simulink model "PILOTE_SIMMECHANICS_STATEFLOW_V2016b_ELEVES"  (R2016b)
settings: Solver=ode45  StartTime=0  StopTime=30  MaxStep=0.05  RelTol=1e-3  EnableMultiTasking=on
undefined symbols (not defined in the file): Bati, coulisseau, deg, kg, m, N, PILOTE_SIMULINK, rad, RootGround, RootPart, s
libraries: mblibv1 x16

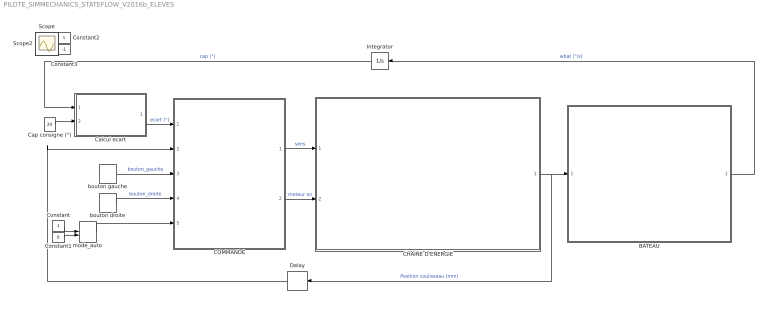
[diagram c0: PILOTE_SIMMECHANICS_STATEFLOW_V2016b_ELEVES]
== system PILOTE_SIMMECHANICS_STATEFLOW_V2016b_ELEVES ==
  BATEAU : Subsystem
  CHAINE D'ENERGIE : Subsystem
  COMMANDE : Stateflow chart  TreatAsAtomicUnit=on
  Calcul ecart : MATLAB Function  TreatAsAtomicUnit=on
  Cap consigne (°) : Constant  Value=20
  Constant : Constant
  Constant1 : Constant  Value=0
  Constant2 : Constant
  Constant3 : Constant  Value=-1
  Delay : Delay  DelayLength=1  SampleTime=0.05
  Integrator : Integrator
  bouton droite : DiscretePulseGenerator  PulseType=Time based  Period=30  PulseWidth=40  PhaseDelay=15
  bouton gauche : DiscretePulseGenerator  PulseType=Time based  Period=30  PulseWidth=40  PhaseDelay=1
  mode_auto : ManualSwitch  CurrentSetting=0
  Scope : Scope
  Scope2 : Scope
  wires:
  Constant/1 -> mode_auto/1
  Constant1/1 -> mode_auto/2
  bouton gauche/1 -> COMMANDE/3(bouton_gauche)  "bouton_gauche"
  bouton droite/1 -> COMMANDE/4(bouton_droite)  "bouton_droite"
  mode_auto/1 -> COMMANDE/5(mode_auto)
  COMMANDE/1(sens_rotation) -> CHAINE D'ENERGIE/1(sens)  "sens"
  COMMANDE/2(moteur_on) -> CHAINE D'ENERGIE/2(moteur_on)  "moteur on"
  BATEAU/1(Out1) -> Integrator/1  "wbat (°/s)"
  Calcul ecart/1(ecart) -> COMMANDE/1(ecart_cap)  "ecart (°)"
  Cap consigne (°)/1 -> Calcul ecart/2(cap_consigne)
  CHAINE D'ENERGIE/1(Pos_coul) -> Delay/1, BATEAU/1(In1)  "Position coulisseau (mm)"
  Integrator/1 -> Calcul ecart/1(cap_mesure)  "cap (°)"
  Constant2/1 -> ?
  Constant3/1 -> ?
  Delay/1 -> COMMANDE/2(pos_coul)

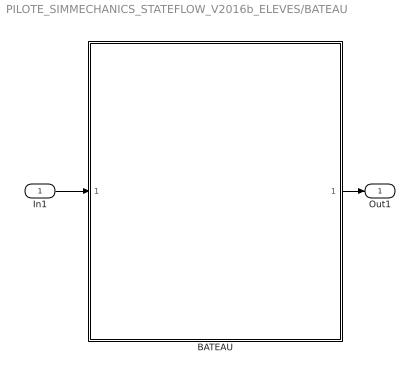
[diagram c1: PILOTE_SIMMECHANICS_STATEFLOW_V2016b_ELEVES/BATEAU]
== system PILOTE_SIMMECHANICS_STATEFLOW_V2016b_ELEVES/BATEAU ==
  In1 : Inport
  BATEAU : MATLAB Function  TreatAsAtomicUnit=on
  Out1 : Outport
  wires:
  In1/1 -> BATEAU/1(pos)
  BATEAU/1(wbat) -> Out1/1

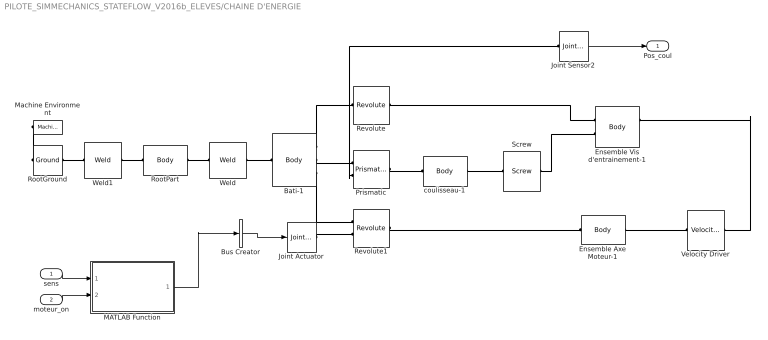
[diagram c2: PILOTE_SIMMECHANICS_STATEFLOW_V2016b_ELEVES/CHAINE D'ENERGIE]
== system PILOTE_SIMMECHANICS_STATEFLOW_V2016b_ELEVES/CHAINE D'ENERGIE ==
  sens : Inport
  moteur_on : Inport  Port=2
  Bati-1 : mblibv1/Bodies/Body  LConnTagsString=CS2  RConnTagsString=CS3|CS4|CS5  UpdateFromCAD=on  PMImportedID=Bati-1  DialogClass=MechanicalBodyBlock  Mass=0.275117  MassUnits=kg  InertiaUnits=kg*m^2  Inertia=[0.00487661,-3.37196e-06,-0.000236406;-3.37196e-06,0.00504829,7.5779e-05;-0.000236406,7.5779e-05,0.000251799]  Shape=Cylinder  ShapeDims=[1 1]  ShapeUnits=m  ShapeUse=false  Density=1  DensityUnits=kg/m^3  DensityUse=false  GraphicsMode=GFXFILE  GraphicsFileName=PILOTE_SIMULINK - Bati-1.STL  BodyColorSelMode=COLORPALETTE  BodyColor=[0.75294 0.75294 0.75294]  AttachedToCS=CS1  CG=Right$CG$[0.280395 0.00767074 -0.0225996]$WORLD$WORLD$m$[0 0 1;1 0 0;0 1 0]$3x3 Transform$rad$WORLD$false$Bati-1::CG(AUTOGEN)  WorkingFrames=Right$CS1$[0 0 0]$WORLD$WORLD$m$[0 0 1;1 0 0;0 1 0]$3x3 Transform$rad$WORLD$false$Bati-1::CS1(AUTOGEN)#Left$CS2$[0.280395 0.00767074 -0.0225996]$WORLD$WORLD$m$[1 0 0;0 1 0;0 0 1]$3x3 Transform$rad$WORLD$true$Bati-1:-:PILOTE_SIMULINK/RootPart::Bati-1(AUTOGEN)#Right$CS3$[0.341 0 -0.015]$WORLD$WORLD$m$[1 0 0;0 1 0;0 0 1]$3x3 Transform$rad$WORLD$true$Bati-1:-:Ensemble Vis d'entrainement-1::Bati-1(AUTO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  CGPos=[0.280395 0.00767074 -0.0225996]  CGRot=[0 0 1;1 0 0;0 1 0]  CS0Pos=[]  CS0Rot=[]  CS1Pos=[0 0 0]  CS1Rot=[0 0 1;1 0 0;0 1 0]  CS2Pos=[0.280395 0.00767074 -0.0225996]  CS2Rot=[1 0 0;0 1 0;0 0 1]  CS3Pos=[0.341 0 -0.015]  CS3Rot=[1 0 0;0 1 0;0 0 1]  CS4Pos=[-0.00290422 0 -0.015]  CS4Rot=[1 0 0;0 1 0;0 0 1]  CS5Pos=[0.371 0.0399019 -0.0121998]  CS5Rot=[1 0 0;0 1 0;0 0 1]  CS6Pos=[0.341 0 -0.015]  CS6Rot=[1 0 0;0 1 0;0 0 1]  CS7Pos=[]  CS7Rot=[]  CS8Pos=[]  CS8Rot=[]  CS9Pos=[]  CS9Rot=[]  CS10Pos=[]  CS10Rot=[]  CS11Pos=[]  CS11Rot=[]  CS12Pos=[]  CS12Rot=[]  CS13Pos=[]  CS13Rot=[]  CS14Pos=[]  CS14Rot=[]  CS15Pos=[]  CS15Rot=[]  CS16Pos=[]  CS16Rot=[]  CS17Pos=[]  CS17Rot=[]  CS18Pos=[]  CS18Rot=[]  CS19Pos=[]  CS19Rot=[]  CS20Pos=[]  CS20Rot=[]
  Bus Creator : BusCreator  Inputs=3
  Ensemble Axe Moteur-1 : mblibv1/Bodies/Body  LConnTagsString=CS2  RConnTagsString=CS1  UpdateFromCAD=on  PMImportedID=Ensemble Axe Moteur-1  DialogClass=MechanicalBodyBlock  Mass=0.330709  MassUnits=kg  InertiaUnits=kg*m^2  Inertia=[5e-05,0,0;0,5e-05,0;0,0,5e-05]  Shape=Cylinder  ShapeDims=[1 1]  ShapeUnits=m  ShapeUse=false  Density=1  DensityUnits=kg/m^3  DensityUse=false  GraphicsMode=GFXFILE  GraphicsFileName=PILOTE_SIMULINK - Ensemble Axe Moteur-1.STL  BodyColorSelMode=COLORPALETTE  BodyColor=[1 0 1]  AttachedToCS=CS1  CG=Right$CG$[0.388245 0.0399019 -0.0121998]$WORLD$WORLD$m$[-1 0 0;0 0.998629 -0.0523416;0 -0.0523416 -0.998629]$3x3 Transform$rad$WORLD$false$Ensemble Axe Moteur-1::CG(AUTOGEN)  WorkingFrames=Right$CS1$[0.373663 0.0782415 -0.0142093]$WORLD$WORLD$m$[-1 0 0;0 0.998629 -0.0523416;0 -0.0523416 -0.998629]$3x3 Transform$rad$WORLD$true$Ensemble Axe Moteur-1::CS1(AUTOGEN)#Left$CS2$[0.371 0.0399019 -0.0121998]$WORLD$WORLD$m$[1 0 0;0 1 0;0 0 1]$3x3 Transform$rad$WORLD$true$Bati-1:-:Ensemble Axe Moteur-1::Ensemble Axe Moteur-1(AUTOGEN)  CGPos=[0.388245 0.0399019 -0.0121998]  CGRot=[-1 0 0;0 0.998629 -0.0523416;0 -0.0523416 -0.998629]  CS0Pos=[]  CS0Rot=[]  CS1Pos=[0.373663 0.0782415 -0.0142093]  CS1Rot=[-1 0 0;0 0.998629 -0.0523416;0 -0.0523416 -0.998629]  CS2Pos=[0.371 0.0399019 -0.0121998]  CS2Rot=[1 0 0;0 1 0;0 0 1]  CS3Pos=[]  CS3Rot=[]  CS4Pos=[]  CS4Rot=[]  CS5Pos=[]  CS5Rot=[]  CS6Pos=[]  CS6Rot=[]  CS7Pos=[]  CS7Rot=[]  CS8Pos=[]  CS8Rot=[]  CS9Pos=[]  CS9Rot=[]  CS10Pos=[]  CS10Rot=[]  CS11Pos=[]  CS11Rot=[]  CS12Pos=[]  CS12Rot=[]  CS13Pos=[]  CS13Rot=[]  CS14Pos=[]  CS14Rot=[]  CS15Pos=[]  CS15Rot=[]  CS16Pos=[]  CS16Rot=[]  CS17Pos=[]  CS17Rot=[]  CS18Pos=[]  CS18Rot=[]  CS19Pos=[]  CS19Rot=[]  CS20Pos=[]  CS20Rot=[]
  Ensemble Vis d'entrainement-1 : mblibv1/Bodies/Body  LConnTagsString=CS2|CS3  RConnTagsString=CS1|CS4  UpdateFromCAD=on  PMImportedID=Ensemble Vis d'entrainement-1  DialogClass=MechanicalBodyBlock  Mass=0.163769  MassUnits=kg  InertiaUnits=kg*m^2  Inertia=[0.00190405,1.37845e-10,-2.6424e-08;1.37845e-10,0.00190406,-8.48302e-09;-2.6424e-08,-8.48302e-09,4.54904e-06]  Shape=Cylinder  ShapeDims=[1 1]  ShapeUnits=m  ShapeUse=false  Density=1  DensityUnits=kg/m^3  DensityUse=false  GraphicsMode=GFXFILE  GraphicsFileName=PILOTE_SIMULINK - Ensemble Vis d'entrainement-1.STL  BodyColorSelMode=COLORPALETTE  BodyColor=[1 0 0]  AttachedToCS=CS1  CG=Right$CG$[0.18733 -5.19925e-07 -0.0149984]$WORLD$WORLD$m$[0 0 -1;-0.606632 -0.794983 0;-0.794983 0.606632 0]$3x3 Transform$rad$WORLD$false$Ensemble Vis d'entrainement-1::CG(AUTOGEN)  WorkingFrames=Right$CS1$[0.361 0 -0.015]$WORLD$WORLD$m$[0 0 -1;-0.606632 -0.794983 0;-0.794983 0.606632 0]$3x3 Transform$rad$WORLD$true$Ensemble Vis d'entrainement-1::CS1(AUTOGEN)#Left$CS2$[0.341 0 -0.015]$WORLD$WORLD$m$[1 0 0;0 1 0;0 0 1]$3x3 Transform$rad$WORLD$true$Bati-1:-:Ensemble Vis d'entrainement-1::Ensemble Vis d'entrainement-1(AUTOGEN)#Right$CS4$[0.341 0 -0.015]$WORLD$WORLD$m$[1 0 0;0 1 0;0 0 1]$3x3 T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  CGPos=[0.18733 -5.19925e-07 -0.0149984]  CGRot=[0 0 -1;-0.606632 -0.794983 0;-0.794983 0.606632 0]  CS0Pos=[]  CS0Rot=[]  CS1Pos=[0.361 0 -0.015]  CS1Rot=[0 0 -1;-0.606632 -0.794983 0;-0.794983 0.606632 0]  CS2Pos=[0.341 0 -0.015]  CS2Rot=[1 0 0;0 1 0;0 0 1]  CS3Pos=[0.0706 0 -0.015]  CS3Rot=[1 0 0;0 1 0;0 0 1]  CS4Pos=[0.341 0 -0.015]  CS4Rot=[1 0 0;0 1 0;0 0 1]  CS5Pos=[]  CS5Rot=[]  CS6Pos=[]  CS6Rot=[]  CS7Pos=[]  CS7Rot=[]  CS8Pos=[]  CS8Rot=[]  CS9Pos=[]  CS9Rot=[]  CS10Pos=[]  CS10Rot=[]  CS11Pos=[]  CS11Rot=[]  CS12Pos=[]  CS12Rot=[]  CS13Pos=[]  CS13Rot=[]  CS14Pos=[]  CS14Rot=[]  CS15Pos=[]  CS15Rot=[]  CS16Pos=[]  CS16Rot=[]  CS17Pos=[]  CS17Rot=[]  CS18Pos=[]  CS18Rot=[]  CS19Pos=[]  CS19Rot=[]  CS20Pos=[]  CS20Rot=[]
  Joint Actuator : mblibv1/Sensors &  Actuators/Joint Actuator  UpdateFromCAD=off  PhysicalDomain=Mechanical  PortType=blob  ActuationStyle=Motion  AngleUnits=rad  ArcVelocityUnits=rad/s  ArcAccelerationUnits=rad/s^2  CoordPositionUnits=m  VelocityUnits=m/s  AccelerationUnits=m/s^2  ForceUnits=N  TorqueUnits=N*m  ActiveIO=on  Width=3  DialogClass=MechanicalActuatorBlock  Primitive=R1  ReferenceFrame=Absolute (World)
  Joint Sensor2 : mblibv1/Sensors &  Actuators/Joint Sensor  UpdateFromCAD=off  PhysicalDomain=Mechanical  PortType=blob  Muxed=off  Pose=off  Angle=off  AngleUnits=deg  ArcVelocity=off  ArcVelocityUnits=deg/s  ArcAcceleration=off  ArcAccelerationUnits=deg/s^2  CoordPosition=on  CoordPositionUnits=mm  Velocity=off  VelocityUnits=m/s  Acceleration=off  AccelerationUnits=m/s^2  Quaternion=on  QuaternionDT=off  QuaternionDDT=off  QuaternionUnits=off  OutputVector=[1]  ActiveIO=on  Width=1  DialogClass=MechanicalSensorBlock  Primitive=P1  Force=off  ForceUnits=N  Torque=on  TorqueUnits=N*m  ReferenceFrame=Absolute (World)  ReactionSensedSide=Base  ReactionReferenceFrame=Absolute (World)  ReactionForce=off  ReactionForceUnits=N  ReactionMoment=off  ReactionMomentUnits=N*m
  MATLAB Function : MATLAB Function  TreatAsAtomicUnit=on
  Machine Environment : mblibv1/Bodies/Machine Environment  PortType=env  PhysicalDomain=Mechanical  DialogTemplateClass=MECH.MachineEnvironment  SyncWhenCopied=off  Gravity=[0 -9.81 0]  GravityUnits=m/s^2  GravityAsSignal=off  Dimensionality=Auto-detect  AnalysisType=Forward dynamics  LinearAssemblyTolerance=1e-3  LinearAssemblyToleranceUnits=m  AngularAssemblyTolerance=1e-3  AngularAssemblyToleranceUnits=rad  ConstraintSolverType=Stabilizing  ConstraintRelTolerance=1e-4  ConstraintAbsTolerance=1e-4  UseRobustSingularityHandling=off  RedundancyAnalysisToleranceType=Automatically select tolerance  RedundancyAnalysisTolerance=1e-14  StatePerturbationType=Fixed  PerturbationSize=1e-5  VisualizeMachine=on  BodyVisualizationType=Use model default body geometries  BodyColorSelMode=Use model default  DefaultBodyColor=[1 0 0]
  Prismatic : mblibv1/Joints/Prismatic  LConnTagsString=__newl0|SA1  RConnTagsString=__newr0  UpdateFromCAD=on  PMImportedID=Bati-1:-:coulisseau-1  NumSAPorts=1  CutJoint=off  MarkAsCut=off  Primitives=prismatic  PrimitiveProps=P1$World$[-1,0,0]$prismatic  DialogClass=JointBlock  P1Axis=[-1,0,0]
  Revolute : mblibv1/Joints/Revolute  LConnTagsString=__newl0  RConnTagsString=__newr0  UpdateFromCAD=on  PMImportedID=Bati-1:-:Ensemble Vis d'entrainement-1  NumSAPorts=0  CutJoint=off  MarkAsCut=off  Primitives=prismatic  PrimitiveProps=R1$World$[1,0,0]$revolute  DialogClass=JointBlock  R1Axis=[1,0,0]
  Revolute1 : mblibv1/Joints/Revolute  LConnTagsString=__newl0|SA1  RConnTagsString=__newr0  UpdateFromCAD=on  PMImportedID=Bati-1:-:Ensemble Axe Moteur-1  NumSAPorts=1  CutJoint=off  MarkAsCut=off  Primitives=prismatic  PrimitiveProps=R1$World$[-1,0,0]$revolute  DialogClass=JointBlock  R1Axis=[-1,0,0]
  RootGround : mblibv1/Bodies/Ground  UpdateFromCAD=on  PMImportedID=RootGround  LeftPortType=env  RightPortType=workingframe  PhysicalDomain=Mechanical  DialogClass=GroundBlock  CoordPosition=[0.246549,0.0167324,-0.0162514]  CoordPositionUnits=m  StateVectorMgrId=2  MachineId=[3 0]  ShowEnvPort=on  ParameterChecksum=[441952517, 4021082612, 3603074577, 143967490]  TopologyChecksum=[1489896608, 3478853089, 1162583120, 1816670376]
  RootPart : mblibv1/Bodies/Body  LConnTagsString=CS3  RConnTagsString=CS2  UpdateFromCAD=on  PMImportedID=PILOTE_SIMULINK/RootPart  DialogClass=MechanicalBodyBlock  Mass=0  MassUnits=kg  InertiaUnits=kg*m^2  Inertia=[0,0,0;0,0,0;0,0,0]  Shape=Cylinder  ShapeDims=[1 1]  ShapeUnits=m  ShapeUse=false  Density=1  DensityUnits=kg/m^3  DensityUse=false  GraphicsMode=MACHINE_DEFAULT  BodyColorSelMode=MACHINE_DEFAULT  BodyColor=[1;0;0]  AttachedToCS=CS1  CG=Right$CG$[0.246549 0.0167324 -0.0162514]$WORLD$WORLD$m$[1 0 0;0 1 0;0 0 1]$3x3 Transform$rad$WORLD$false$PILOTE_SIMULINK/RootPart::CG(AUTOGEN)  WorkingFrames=Right$CS1$[0 0 0]$WORLD$WORLD$m$[1 0 0;0 1 0;0 0 1]$3x3 Transform$rad$WORLD$false$PILOTE_SIMULINK/RootPart::CS1(AUTOGEN)#Right$CS2$[0.280395 0.00767074 -0.0225996]$WORLD$WORLD$m$[1 0 0;0 1 0;0 0 1]$3x3 Transform$rad$WORLD$true$Bati-1:-:PILOTE_SIMULINK/RootPart::PILOTE_SIMULINK/RootPart(AUTOGEN)#Left$CS3$[0.246549 0.0167324 -0.0162514]$WORLD$WORLD$m$[1 0 0;0 1 0;0 0 1]$3x3 Transform$rad$WORLD$true$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  CGPos=[0.246549 0.0167324 -0.0162514]  CGRot=[1 0 0;0 1 0;0 0 1]  CS0Pos=[]  CS0Rot=[]  CS1Pos=[0 0 0]  CS1Rot=[1 0 0;0 1 0;0 0 1]  CS2Pos=[0.280395 0.00767074 -0.0225996]  CS2Rot=[1 0 0;0 1 0;0 0 1]  CS3Pos=[0.246549 0.0167324 -0.0162514]  CS3Rot=[1 0 0;0 1 0;0 0 1]  CS4Pos=[]  CS4Rot=[]  CS5Pos=[]  CS5Rot=[]  CS6Pos=[]  CS6Rot=[]  CS7Pos=[]  CS7Rot=[]  CS8Pos=[]  CS8Rot=[]  CS9Pos=[]  CS9Rot=[]  CS10Pos=[]  CS10Rot=[]  CS11Pos=[]  CS11Rot=[]  CS12Pos=[]  CS12Rot=[]  CS13Pos=[]  CS13Rot=[]  CS14Pos=[]  CS14Rot=[]  CS15Pos=[]  CS15Rot=[]  CS16Pos=[]  CS16Rot=[]  CS17Pos=[]  CS17Rot=[]  CS18Pos=[]  CS18Rot=[]  CS19Pos=[]  CS19Rot=[]  CS20Pos=[]  CS20Rot=[]
  Screw : mblibv1/Joints/Screw  LConnTagsString=__newl0  RConnTagsString=__newr0  UpdateFromCAD=off  NumSAPorts=0  CutJoint=off  MarkAsCut=off  Primitives=prismatic  PrimitiveProps=R1$World$[1 0 0]$revolute  DialogClass=ScrewJointBlock  Pitch=3  Units=mm  R1Axis=[1 0 0]
  Velocity Driver : mblibv1/Constraints &  Drivers/Velocity Driver  LConnTagsString=__newl0  RConnTagsString=__newr0  UpdateFromCAD=off  DialogClass=ConstantVelocityConstraint  NumSAPorts=0  Unit_V=m/s  Unit_Omega=rad/s  Coef_V_Base=[1 0 0]  Csys_V_Base=World  Coef_Omega_Base=[1 0 0]  Csys_Omega_Base=World  Coef_V_Follower=[1 0 0]  Csys_V_Follower=World  Coef_Omega_Follower=[71/20 0 0]  Csys_Omega_Follower=World
  Weld : mblibv1/Joints/Weld  LConnTagsString=__newl0  RConnTagsString=__newr0  UpdateFromCAD=on  PMImportedID=Bati-1:-:PILOTE_SIMULINK/RootPart  NumSAPorts=0  CutJoint=off  MarkAsCut=off  Primitives=weld  PrimitiveProps=W$WORLD$[0.57735,0.57735,0.57735]$weld  DialogClass=JointBlock  WAxis=[0.57735,0.57735,0.57735]
  Weld1 : mblibv1/Joints/Weld  LConnTagsString=__newl0  RConnTagsString=__newr0  UpdateFromCAD=on  PMImportedID=PILOTE_SIMULINK/RootPart:-:RootGround  NumSAPorts=0  CutJoint=off  MarkAsCut=off  Primitives=weld  PrimitiveProps=W$WORLD$[0.57735,0.57735,0.57735]$weld  DialogClass=JointBlock  WAxis=[0.57735,0.57735,0.57735]
  coulisseau-1 : mblibv1/Bodies/Body  LConnTagsString=CS2  RConnTagsString=CS3  UpdateFromCAD=on  PMImportedID=coulisseau-1  DialogClass=MechanicalBodyBlock  Mass=0.145203  MassUnits=kg  InertiaUnits=kg*m^2  Inertia=[0.00230468,3.3163e-09,1.1845e-07;3.3163e-09,0.00230538,-1.12769e-06;1.1845e-07,-1.12769e-06,9.33916e-06]  Shape=Cylinder  ShapeDims=[1 1]  ShapeUnits=m  ShapeUse=false  Density=1  DensityUnits=kg/m^3  DensityUse=false  GraphicsMode=GFXFILE  GraphicsFileName=PILOTE_SIMULINK - coulisseau-1.STL  BodyColorSelMode=COLORPALETTE  BodyColor=[0 0.75294 0]  AttachedToCS=CS1  CG=Right$CG$[0.185 3.88471e-06 -0.0148643]$World$World$m$[0 0 1;1 0 0;0 1 0]$3x3 Transform$rad$WORLD$false$coulisseau-1::CG(AUTOGEN)  WorkingFrames=Right$CS1$[0.185 0.0253055 -0.0241096]$WORLD$WORLD$m$[0 0 1;1 0 0;0 1 0]$3x3 Transform$rad$WORLD$false$coulisseau-1::CS1(AUTOGEN)#Left$CS2$[0.031 0 -0.015]$WORLD$WORLD$m$[1 0 0;0 1 0;0 0 1]$3x3 Transform$rad$WORLD$true$Bati-1:-:coulisseau-1::coulisseau-1(AUTOGEN)#Right$CS3$[0.0706 0 -0.015]$WORLD$WORLD$m$[1 0 0;0 1 0;0 0 1]$3x3 Transform$rad$WORLD$true$Ensemble Vis d'entrainement-1:-:coulisseau-1: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  CGPos=[0.185 3.88471e-06 -0.0148643]  CGRot=[0 0 1;1 0 0;0 1 0]  CS0Pos=[]  CS0Rot=[]  CS1Pos=[0.185 0.0253055 -0.0241096]  CS1Rot=[0 0 1;1 0 0;0 1 0]  CS2Pos=[0.031 0 -0.015]  CS2Rot=[1 0 0;0 1 0;0 0 1]  CS3Pos=[0.0706 0 -0.015]  CS3Rot=[1 0 0;0 1 0;0 0 1]  CS4Pos=[]  CS4Rot=[]  CS5Pos=[]  CS5Rot=[]  CS6Pos=[]  CS6Rot=[]  CS7Pos=[]  CS7Rot=[]  CS8Pos=[]  CS8Rot=[]  CS9Pos=[]  CS9Rot=[]  CS10Pos=[]  CS10Rot=[]  CS11Pos=[]  CS11Rot=[]  CS12Pos=[]  CS12Rot=[]  CS13Pos=[]  CS13Rot=[]  CS14Pos=[]  CS14Rot=[]  CS15Pos=[]  CS15Rot=[]  CS16Pos=[]  CS16Rot=[]  CS17Pos=[]  CS17Rot=[]  CS18Pos=[]  CS18Rot=[]  CS19Pos=[]  CS19Rot=[]  CS20Pos=[]  CS20Rot=[]
  Pos_coul : Outport
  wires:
  Joint Sensor2/1 -> Pos_coul/1
  moteur_on/1 -> MATLAB Function/2(moteur_on)
  sens/1 -> MATLAB Function/1(sens)
  Bus Creator/1 -> Joint Actuator/1
  MATLAB Function/1(wmot) -> Bus Creator/2
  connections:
  Weld/RConn1 -- Bati-1/LConn1
  Bati-1/RConn1 -- Revolute/LConn1
  Bati-1/RConn2 -- Prismatic/LConn1
  Bati-1/RConn3 -- Revolute1/LConn1
  Ensemble Axe Moteur-1/RConn1 -- Velocity Driver/LConn1
  Screw/LConn1 -- Ensemble Vis d'entrainement-1/LConn2
  RootGround/LConn1 -- Machine Environment/RConn1
  Prismatic/RConn1 -- coulisseau-1/LConn1
  RootGround/RConn1 -- Weld1/LConn1
  Weld1/RConn1 -- RootPart/LConn1
  RootPart/RConn1 -- Weld/LConn1
  Screw/RConn1 -- coulisseau-1/RConn1
  Revolute1/RConn1 -- Ensemble Axe Moteur-1/LConn1
  Revolute/RConn1 -- Ensemble Vis d'entrainement-1/LConn1
  Velocity Driver/RConn1 -- Ensemble Vis d'entrainement-1/RConn1
  Joint Sensor2/LConn1 -- Prismatic/LConn2
  Joint Actuator/RConn1 -- Revolute1/LConn2

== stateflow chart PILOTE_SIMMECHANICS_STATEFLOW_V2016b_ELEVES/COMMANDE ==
  state AUTO
    state SENS [parallel]
      state AUTO_ARRET
      state AUTO_GAUCHE
        sens_rotation=1;
      state AUTO_DROITE
        sens_rotation=0;
      (default) -> AUTO_ARRET
      AUTO_ARRET -> AUTO_GAUCHE : [after(40,sec)]
      AUTO_DROITE -> AUTO_ARRET
      AUTO_GAUCHE -> AUTO_DROITE
    state MOTEUR [parallel]
      state MOTEUR_ON
        moteur_on=1;
      state MOTEUR_OFF
        moteur_on=0;
      (default) -> MOTEUR_OFF
      MOTEUR_OFF -> MOTEUR_ON : [in(SENS.AUTO_GAUCHE)  | in(SENS.AUTO_DROITE) ]
      MOTEUR_ON -> MOTEUR_OFF : [in(SENS.AUTO_ARRET) ]
  state MANUEL
    state SENS [parallel]
      state ARRET
      state GAUCHE
        sens_rotation=1;
      state DROITE
        sens_rotation=0;
      (default) -> ARRET
      ARRET -> GAUCHE : [after(40,sec)]
      DROITE -> ARRET
      GAUCHE -> DROITE
    state MOTEUR [parallel]
      state MOTEUR_OFF
        moteur_on=0;
      state MOTEUR_ON
        moteur_on=1;
      (default) -> MOTEUR_OFF
      MOTEUR_OFF -> MOTEUR_ON : [in(SENS.GAUCHE) | in(SENS.DROITE)]
      MOTEUR_ON -> MOTEUR_OFF : [in(SENS.ARRET)]
  (default) -> MANUEL
  MANUEL -> AUTO : [mode_auto==1]
  AUTO -> MANUEL : [mode_auto==0]
  data: ecart_cap input; sens_rotation output double; moteur_on output double; pos_coul input; bouton_gauche input; bouton_droite input; mode_auto input

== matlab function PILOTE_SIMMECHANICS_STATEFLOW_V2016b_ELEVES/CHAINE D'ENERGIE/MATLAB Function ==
function wmot = fcn(sens,moteur_on)
%#codegen

if moteur_on == 1
    if sens == 0
        wmot = 1; %completer la vitesse wmot en rd/s (positive)
    else
        wmot = -1; %completer la vitesse wmot en rd/s (negative)
    end
else
    wmot = 0;
end

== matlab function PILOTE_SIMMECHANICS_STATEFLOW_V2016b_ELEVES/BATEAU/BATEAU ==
function wbat = fcn(pos)
%#codegen

wbat = pos; %completer l'equation wbat = f (pos)

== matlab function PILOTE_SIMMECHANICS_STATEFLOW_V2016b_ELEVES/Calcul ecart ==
function ecart = fcn(cap_mesure,cap_consigne)
%#codegen

ecart = cap_consigne-cap_mesure;
